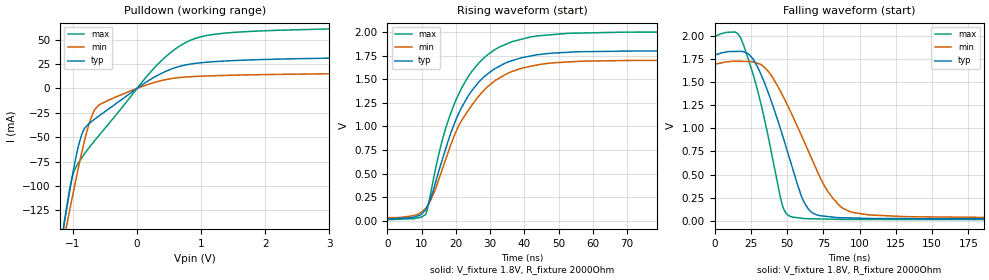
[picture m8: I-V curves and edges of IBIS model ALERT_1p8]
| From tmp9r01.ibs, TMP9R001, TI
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|   Model
[Model]   ALERT_1p8
Model_type   Open_drain
Polarity   Non-Inverting
Vmeas = 0.9
Vref = 1.8
Cref = 1pF
Rref = 2000
|   typ   min   max
C_comp   1.523pF   1.378pF   1.601pF
[Voltage Range]   1.8   1.7   2
[Temperature Range]   25   125   -40
[Pullup Reference]   1.8   1.7   2
[Pulldown Reference]   -0   0   0
[Power Clamp Reference]   1.8   1.7   2
[GND Clamp Reference]   0   0   0
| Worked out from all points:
|   slope of the pulldown table from 0 to 0.27 V, typ, clamps not added: 23.5 ohm
|   falling waveform, V_fixture 1.8V, R_fixture 2000Ohm: 20-80 % time 21.9ns typ, 29.6ns min, 17.2ns max; typ from 1.8 V to 0.019 V
|   rising waveform, V_fixture 1.8V, R_fixture 2000Ohm: 20-80 % time 12.3ns typ, 13.5ns min, 11.8ns max; typ from 0.019 V to 1.8 V
[Pulldown]
|   Voltage   I(typ)   I(min)   I(max)
-1.8V     -422.9mA   -392.3mA   -467.2mA
-1.195V   -162.2mA   -173.7mA   -163.7mA
-1.125V   -133.8mA   -149.5mA   -131.9mA
-1.049V   -104.4mA   -124.2mA   -102mA
-995.4mV  -84.52mA   -106.5mA   -87.15mA
-865.8mV  -47.52mA   -66.48mA   -71.31mA
-747mV    -35.93mA   -35.56mA   -60.55mA
-595.8mV  -28.29mA   -16.94mA   -48.32mA
273.6mV   11.64mA    6.12mA     21.26mA
743.4mV   23.8mA     11.54mA    46.41mA
1.445V    28.28mA    13.4mA     56.98mA
3.6V      31.71mA    15.37mA    61.83mA
[Ramp]
R_load = 2000
|   typ   min   max
dV/dt_r   1.06867/1.22291e-08   1.00015/1.34094e-08   1.19298/1.18153e-08
dV/dt_f   1.06863/2.18937e-08   0.99995/2.95738e-08   1.19297/1.72166e-08
[Falling Waveform]
V_fixture = 1.8V
V_fixture_min = 1.7V
V_fixture_max = 2V
R_fixture = 2000Ohm
C_fixture = 0F
|   Time   V(typ)   V(min)   V(max)
0s        1.8V       1.7V       2V
13.57ns   1.83V      1.724V     2.04V
18.74ns   1.831V     1.723V     1.948V
30.97ns   1.618V     1.694V     1.325V
46.4ns    944.2mV    1.369V     185.9mV
52ns      657.8mV    1.192V     48.65mV
65.55ns   109.9mV    721.6mV    22.06mV
78.48ns   44.97mV    308.6mV    17.76mV
94.13ns   30.25mV    95.7mV     14.81mV
300ns     18.94mV    33.42mV    11.72mV
[Rising Waveform]
V_fixture = 1.8V
V_fixture_min = 1.7V
V_fixture_max = 2V
R_fixture = 2000Ohm
C_fixture = 0F
|   Time   V(typ)   V(min)   V(max)
0s        18.88mV    33.08mV    11.71mV
11.09ns   115.3mV    127.4mV    64.64mV
13.82ns   375.1mV    315.2mV    507.7mV
16.88ns   746.2mV    635.2mV    963.1mV
19.68ns   1.04V      914.2mV    1.25V
22.99ns   1.286V     1.135V     1.491V
31.6ns    1.615V     1.489V     1.818V
41.51ns   1.744V     1.634V     1.945V
71.15ns   1.798V     1.698V     1.998V
300ns     1.8V       1.7V       2V
